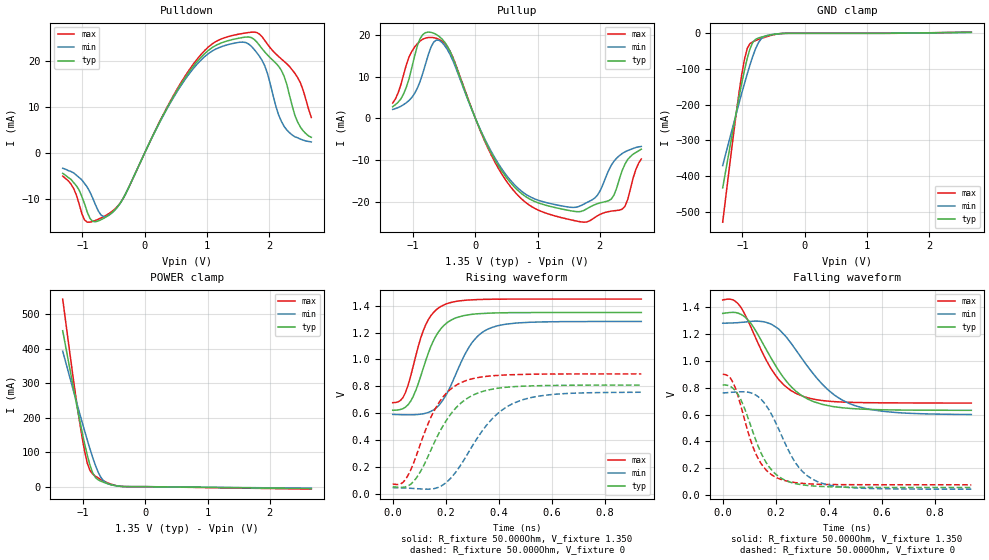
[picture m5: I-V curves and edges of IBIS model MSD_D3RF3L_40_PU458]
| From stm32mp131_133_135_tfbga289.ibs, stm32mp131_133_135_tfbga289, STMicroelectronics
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[Model] MSD_D3RF3L_40_PU458
Model_type   I/O
C_comp 2.396pF   2.311pF   2.520pF
Vinh = 810.000mV
Vinl = 540.000mV
Vmeas = 675.000mV
Vref = 675.000mV
[Model Spec]
Vinh   810.000mV   777.000mV   860.000mV
Vinl   540.000mV   507.000mV   590.000mV
Vmeas   675.000mV   642.000mV   725.000mV
Vref   675.000mV   642.000mV   725.000mV
[Receiver Thresholds]
Vth   =  0.675V
Vth_min  =  0.6615V
Vth_max  =  0.6885V
Vinh_ac  =  0.160V
Vinh_dc  =  0.090V
Vinl_ac  = -0.160V
Vinl_dc  = -0.090V
Tslew_ac =  5.000ns |Not specified, so set to high value
Threshold_sensitivity = 0.50
Reference_supply Pullup_ref
[Temperature Range]   25.000   125.000   -40.000
[Voltage Range]   1.350V   1.283V   1.450V
[GND Clamp Reference]   0.00V   0.00V   0.00V
[Pulldown Reference]   0.00V   0.00V   0.00V
[POWER Clamp Reference]   1.350V   1.283V   1.450V
[Pullup Reference]   1.350V   1.283V   1.450V
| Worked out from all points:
|   slope of the pulldown table from 0 to 0.203 V, typ, clamps not added: 35.6 ohm
|   slope of the pullup table from 0 to 0.203 V, typ, clamps not added: 29.7 ohm
|   GND clamp passes 1 mA (typ) near -0.40 V on its own axis
|   POWER clamp passes 1 mA (typ) near -0.41 V on its own axis
|   rising waveform, R_fixture 50.000Ohm, V_fixture 1.350: 20-80 % time 85.8ps typ, 108ps min, 72.8ps max; typ from 0.621 V to 1.35 V
|   rising waveform, R_fixture 50.000Ohm, V_fixture 0: 20-80 % time 133ps typ, 159ps min, 113ps max; typ from 0.051 V to 0.809 V
|   falling waveform, R_fixture 50.000Ohm, V_fixture 1.350: 20-80 % time 146ps typ, 175ps min, 127ps max; typ from 1.35 V to 0.632 V
|   falling waveform, R_fixture 50.000Ohm, V_fixture 0: 20-80 % time 97.4ps typ, 116ps min, 84.4ps max; typ from 0.822 V to 0.057 V
[GND Clamp]
-1.318V   -433.3mA   -370.7mA   -529.5mA
-1.142V   -261mA     -253.1mA   -280.7mA
-1.055V   -178.6mA   -195.5mA   -165.6mA
-1.011V   -139.4mA   -167.5mA   -114.5mA
-966.7mV  -102.7mA   -139.9mA   -71.66mA
-922.7mV  -69.78mA   -113.4mA   -42.02mA
-878.8mV  -43.16mA   -88.12mA   -28.62mA
-790.9mV  -17.05mA   -44.03mA   -20.47mA
-703mV    -10.93mA   -16.1mA    -14.81mA
-527.3mV  -3.949mA   -3.336mA   -5.27mA
-307.6mV  -123uA     -180.2uA   -110uA
2.68V     2.885mA    2.451mA    3.413mA
[Power Clamp]
-1.33V    452.7mA    393.2mA    544.5mA
-1.111V   242.2mA    247.6mA    251.2mA
-1.023V   162.6mA    190.6mA    148.4mA
-978.8mV  125.5mA    162.7mA    103.9mA
-934.9mV  91.37mA    135.4mA    68.38mA
-890.9mV  62mA       109.1mA    46.75mA
-847mV    39.66mA    84.12mA    36.27mA
-803mV    26.32mA    61.3mA     30.18mA
-715.1mV  15.66mA    26.54mA    20.71mA
-671.2mV  12.44mA    16.45mA    16.56mA
-407.6mV  911.2uA    1.194mA    1.103mA
2.668V    -5.686mA   -4.559mA   -7.317mA
[Pulldown]
-1.318V   -4.4mA     -3.3mA     -5mA
-922.7mV  -12.81mA   -7.4mA     -14.98mA
-703mV    -14.45mA   -13.41mA   -14.07mA
-571.2mV  -13.38mA   -13.45mA   -13.08mA
-351.5mV  -9.986mA   -9.957mA   -9.956mA
747mV     18.13mA    17.69mA    18.58mA
1.098V    22.94mA    22.18mA    23.73mA
1.582V    25.03mA    24.01mA    25.9mA
1.889V    22.57mA    20.05mA    25.16mA
2.241V    16.67mA    5.8mA      19.86mA
2.461V    6.7mA      3.3mA      16.3mA
2.68V     3.4mA      2.4mA      7.7mA
[Pullup]
-1.33V    2.8mA      2.152mA    3.679mA
-1.155V   5.9mA      3.31mA     10.51mA
-978.8mV  14.9mA     5.977mA    17.15mA
-715.1mV  20.68mA    17.11mA    19.47mA
-451.5mV  17.38mA    16.56mA    17.25mA
251.5mV   -8.249mA   -7.87mA    -8.718mA
866.7mV   -19.34mA   -18.75mA   -20.85mA
1.702V    -22.36mA   -20.93mA   -24.89mA
1.965V    -20.49mA   -18.41mA   -23.39mA
2.185V    -19.39mA   -11.26mA   -22.29mA
2.361V    -12.5mA    -8.438mA   -21.82mA
2.668V    -7.4mA     -6.748mA   -9.748mA
[Ramp]
R_load=50.000Ohm
dV/dt_r   441.270mV/109.500ps  419.292mV/133.500ps  473.775mV/93.000ps
dV/dt_f   441.270mV/122.500ps  419.292mV/147.000ps  473.775mV/106.000ps
[Rising waveform]
R_fixture=50.000Ohm
V_fixture=1.350
V_fixture_min=1.283
V_fixture_max=1.450
0s        621.3mV    590.5mV    678.2mV
39ps      633.9mV    588.1mV    717.1mV
68ps      689.7mV    587.6mV    877.2mV
96ps      817.4mV    589.9mV    1.095V
125ps     993.9mV    599.8mV    1.261V
163ps     1.175V     637.5mV    1.368V
202ps     1.269V     736.9mV    1.414V
298ps     1.336V     1.122V     1.444V
374ps     1.346V     1.238V     1.449V
938ps     1.35V      1.283V     1.45V
[Rising waveform]
R_fixture=50.000Ohm
V_fixture=0
0s        51.26mV    44.18mV    71.37mV
39ps      47.26mV    42.38mV    84.36mV
87ps      110.9mV    37.55mV    271.4mV
135ps     285.3mV    33.43mV    528.5mV
173ps     445mV      47.67mV    673.9mV
259ps     678mV      220.3mV    828.6mV
355ps     770.1mV    512.4mV    874.3mV
460ps     797.5mV    677.2mV    886.9mV
614ps     806.5mV    740.9mV    891.5mV
938ps     809.3mV    755.5mV    892.2mV
[Falling waveform]
R_fixture=50.000Ohm
V_fixture=1.350
V_fixture_min=1.283
V_fixture_max=1.450
0s        1.355V     1.282V     1.455V
48ps      1.362V     1.285V     1.445V
96ps      1.305V     1.293V     1.298V
192ps     990mV      1.264V     914.6mV
230ps     874.9mV    1.2V       822.9mV
288ps     756.7mV    1.049V     748.2mV
393ps     669.3mV    793.1mV    701.6mV
499ps     644mV      667.3mV    690.9mV
652ps     634.8mV    616.2mV    687.6mV
938ps     632.3mV    600.9mV    686.3mV
[Falling waveform]
R_fixture=50.000Ohm
V_fixture=0
0s        821.6mV    761.5mV    900.6mV
29ps      810.6mV    765.9mV    873mV
48ps      778.2mV    768.7mV    797.8mV
77ps      673.3mV    770.6mV    602.9mV
125ps     409.2mV    745.7mV    307.6mV
163ps     245.6mV    670.4mV    188.6mV
211ps     138.7mV    493.1mV    123.5mV
288ps     80.46mV    205.2mV    89.7mV
374ps     64.06mV    88.4mV     80.07mV
938ps     56.82mV    44.18mV    76.96mV
